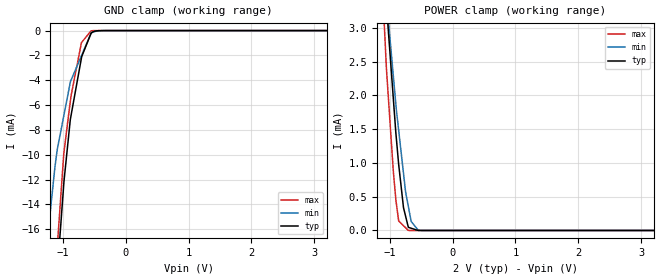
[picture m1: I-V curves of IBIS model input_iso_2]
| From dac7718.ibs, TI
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|   input_iso_2 Model
[Model]   input_iso_2
Model_type   Input
Vinl = 0.3
Vinh = 1.5
|   typ   min   max
|   (Nom PVT)   (Fast PVT)   (Slow PVT)
|C_comp from frequency method(F=50MHz)
|Average
|C_comp   4.106e-12   4.082e-12   4.617e-12
|C_comp from LC tank method(L=1nH)
|Resonant Frequency(Hz)   3.28e9   3.34e9   3.22e9
C_comp   2.357e-12   2.273e-12   2.445e-12
| Where nom  PVT is Nominal Process,  2V,  33C
|   Fast PVT is Strong Process,   2.2V,  -40C
|   Slow PVT is Weak Process,   1.8V,  113C
[Voltage Range]   2   1.8   2.2
|Ambient Temperature   25   85   -40
|Junction Temperature
[Temperature Range]   33   113   -40
[Power Clamp Reference]   2   1.8   2.2
[GND Clamp Reference]   0   0   0
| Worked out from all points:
|   GND clamp passes 1 mA (typ) near -0.61 V on its own axis
|   POWER clamp passes 1 mA (typ) near -0.86 V on its own axis
[GND Clamp]
|   Voltage   I(typ)   I(min)   I(max)
-2V       -111.1mA   -62.07mA   -124.7mA
-1.245V   -32.44mA   -16.8mA    -32.52mA
-1.125V   -22.32mA   -10.95mA   -20.81mA
-1.089V   -19.5mA    -9.586mA   -17.43mA
-985.6mV  -12.39mA   -6.886mA   -9.937mA
-882mV    -7.205mA   -4.18mA    -5.719mA
-864.6mV  -6.701mA   -3.936mA   -5.128mA
-704mV    -2.199mA   -2.028mA   -968.2uA
-550mV    -203.6uA   -198.7uA   -18.46uA
-486mV    -44.96uA   -72.68uA   -2.626uA
-374mV    -2.025uA   -7.529uA   -26.19nA
4V        0A         0A         0A
[POWER Clamp]
|   Voltage   I(typ)   I(min)   I(max)
-2V       21.32mA    17.9mA     23.92mA
-1.164V   5.377mA    4.994mA    4.513mA
-1.054V   3.44mA     3.468mA    2.422mA
-1.028V   3.03mA     3.172mA    2.055mA
-941.6mV  1.938mA    2.275mA    861.1uA
-902mV    1.438mA    1.864mA    449.4uA
-858mV    979.9uA    1.484mA    142.3uA
-780mV    334uA      838.5uA    70.33uA
-704mV    46.8uA     356.2uA    194.3nA
-658.8mV  33.13uA    133.5uA    137.4nA
-513mV    62.52nA    2.577uA    0A
4V        0A         0A         0A
